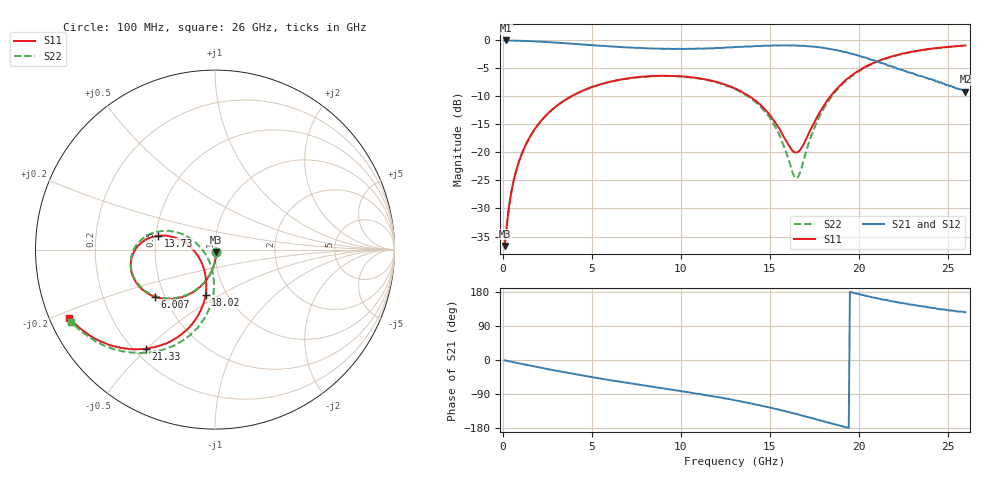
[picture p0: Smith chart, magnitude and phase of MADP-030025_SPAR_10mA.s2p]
!Mean
# HZ S DB R 50
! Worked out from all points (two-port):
!   400 points, 100 MHz to 26 GHz, reference 50 ohm
!   highest |S21| = -0.05 dB at 164.9 MHz (marker M1); lowest = -9.2 dB at 26 GHz (marker M2)
!   |S21| within 3 dB of the highest: start of sweep to 20.33 GHz
!   lowest |S11| = -36.7 dB at 100 MHz (marker M3), VSWR 1.03, Z = 50.6 - j1.34 ohm
!   |S11| at or under -10 dB: start of sweep to 3.851 GHz; 13.87 GHz to 18.41 GHz (4.548 GHz wide, 28.2 % of centre)
!   |S22| runs from -36.7 to -0.9 dB; largest |S21 - S12| = 0.0057
!   S11 on the Smith chart (normalised r, x): 100 MHz: 1.01, -0.03; 6.007 GHz: 0.44, -0.28; 13.73 GHz: 0.51, +0.09; 18.02 GHz: 0.80, -0.43; 21.33 GHz: 0.25, -0.50; 26 GHz: 0.06, -0.22
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1e8  -36.68 -64.4  -0.06 -0.7  -0.05 -0.8  -36.72 -64.2
1.6491e8  -34.93 -70.1  -0.05 -1.5  -0.06 -1.5  -34.90 -70.9
3.5965e8  -29.42 -81.2  -0.07 -3.5  -0.07 -3.5  -29.44 -81.0
6.193e8  -24.88 -87.9  -0.08 -6.1  -0.09 -6.1  -24.91 -88.3
1.3333e9  -18.33 -98.7  -0.14 -12.9  -0.15 -12.9  -18.39 -98.8
2.6316e9  -12.77 -112.5  -0.36 -25.0  -0.36 -24.9  -12.81 -112.9
4.4491e9  -9.06 -129.1  -0.76 -40.6  -0.76 -40.6  -9.09 -129.8
6.007e9  -7.43 -141.8  -1.10 -53.1  -1.11 -53.0  -7.45 -142.7
8.7982e9  -6.36 -162.1  -1.48 -73.5  -1.49 -73.5  -6.39 -163.6
1.1005e10  -6.77 -176.9  -1.49 -89.3  -1.49 -89.4  -6.83 -179.3
1.3082e10  -8.66 169.8  -1.22 -106.6  -1.24 -106.6  -8.76 165.6
1.3732e10  -9.75 166.3  -1.14 -112.5  -1.16 -112.6  -9.93 161.3
1.5095e10  -13.70 164.2  -0.98 -126.6  -0.97 -126.5  -14.27 154.8
1.6458e10  -20.03 -152.0  -0.97 -142.0  -0.98 -142.1  -24.55 -154.9
1.6653e10  -19.76 -138.3  -0.99 -144.6  -0.99 -144.6  -24.02 -130.3
1.7367e10  -15.51 -107.7  -1.12 -153.4  -1.12 -153.3  -16.80 -93.9
1.8016e10  -11.79 -101.8  -1.36 -161.7  -1.38 -161.7  -12.32 -91.9
1.9379e10  -6.82 -108.1  -2.21 -178.6  -2.20 -178.6  -6.99 -102.5
2.1326e10  -3.45 -124.9  -4.08 159.6  -4.04 159.8  -3.51 -121.3
2.1716e10  -3.04 -128.0  -4.51 156.3  -4.51 156.3  -3.09 -124.7
2.4053e10  -1.53 -144.4  -6.89 137.6  -6.86 138.2  -1.54 -142.3
2.6e10  -0.94 -155.0  -9.20 125.9  -9.08 125.9  -0.94 -153.3
